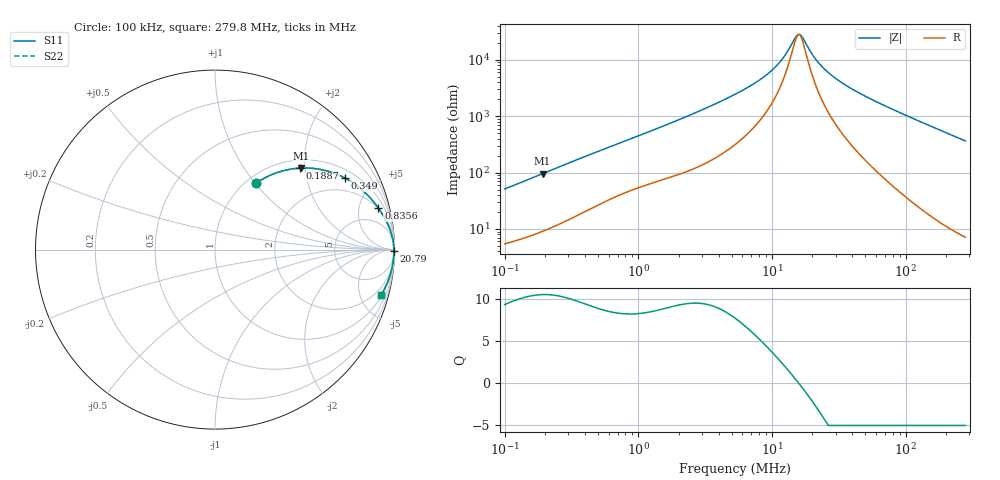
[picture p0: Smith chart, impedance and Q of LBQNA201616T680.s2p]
! LBQNA201616T680  S-PARAMETER MODEL  ( General Type )
! Model Generated by TAIYO YUDEN Corporation (http://www.ty-top.com)
! Version 1.0
! TAIYO YUDEN Control No. 191025NI43SB-FBB
! Copyright(c) 2019 TAIYO YUDEN CO.,LTD. All Rights Reserved.
! Product Description (link to TY-COMPAS)
! https://ds.yuden.co.jp/TYCOMPAS/or/detail?pn=LBQNA201616T680K&u=M
! Products Name : Inductors
! Characteristics :
!  Inductance : 68 uH , SRF(min) : 10 MHz , DC Resistance(max) : 3.9 Ohm
!  Rated Current : Saturation :90 mA , Temp Rise : 110 mA (20 degC)
!  Case Size : 2.0 x 1.6 / 0.079 x 0.063 [mm/inch] , Thickness : 1.6 / 0.063 [mm/inch]
!  (Conditions: Temperature = 25 degC , DC Bias Current/Voltage = 0A / 0V)
! External Node Assignments :
!  1  o---GGG---o  2
! GND o---------o GND
! Frequency Range : 0.1MHz  -  279.750408MHz  [ 402 STEP ]
# MHz S RI R 50
! Freq[MHz].  S11 Real  S11 Imag  S21 Real  S21 Imag  S12 Real  S12 Imag  S22 Real  S22 Imag
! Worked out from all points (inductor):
!   401 points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, 100 kHz to 279.8 MHz, reference 50 ohm
!   read as one part in series: L = 80 uH near 104 kHz
!   highest Q = 10.5 at 192.5 kHz (marker M1), where L = 78.9 uH
!   self-resonance near 15.75 MHz
!   S11 on the Smith chart (normalised r, x): 100 kHz: 1.11, +1.01; 188.7 kHz: 1.18, +1.87; 349 kHz: 1.35, +3.37; 835.6 kHz: 1.92, +7.54; 20.79 MHz: open; 279.8 MHz: 1.14, -7.27
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0.1  0.2294 0.3703  0.7706 -0.3703  0.7706 -0.3703  0.2294 0.3703
0.188687  0.4721 0.4539  0.5279 -0.4539  0.5279 -0.4539  0.4721 0.4539
0.192468  0.4808 0.4544  0.5192 -0.4544  0.5192 -0.4544  0.4808 0.4544
0.349033  0.7221 0.3996  0.2779 -0.3996  0.2779 -0.3996  0.7221 0.3996
0.377863  0.7479 0.385  0.2521 -0.385  0.2521 -0.385  0.7479 0.385
0.835625  0.9108 0.2307  0.0892 -0.2307  0.0892 -0.2307  0.9108 0.2307
1.427803  0.9585 0.1502  0.0415 -0.1502  0.0415 -0.1502  0.9585 0.1502
5.289144  0.9931 0.0402  0.00686 -0.0402  0.00686 -0.0402  0.9931 0.0402
7.710934  0.9951 0.0239  0.00494 -0.0239  0.00494 -0.0239  0.9951 0.0239
10.17991  0.9958 0.0141  0.00415 -0.0141  0.00415 -0.0141  0.9958 0.0141
12.17016  0.9962 0.00827  0.00382 -0.00827  0.00382 -0.00827  0.9962 0.00827
14.84108  0.9964 0.00209  0.00359 -0.00209  0.00359 -0.00209  0.9964 0.00209
15.7513  0.9965 0.00025  0.00354 -0.00025  0.00354 -0.00025  0.9965 0.00025
17.05234  0.9965 -0.0022  0.00349 0.0022  0.00349 0.0022  0.9965 -0.0022
19.9857  0.9965 -0.00718  0.00345 0.00718  0.00345 0.00718  0.9965 -0.00718
20.79473  0.9965 -0.00845  0.00345 0.00845  0.00345 0.00845  0.9965 -0.00845
25.35844  0.9965 -0.015  0.00354 0.015  0.00354 0.015  0.9965 -0.015
32.82031  0.9961 -0.0246  0.00385 0.0246  0.00385 0.0246  0.9961 -0.0246
46.90804  0.9951 -0.0406  0.00488 0.0406  0.00488 0.0406  0.9951 -0.0406
75.51853  0.9917 -0.0703  0.00828 0.0703  0.00828 0.0703  0.9917 -0.0703
148.2617  0.976 -0.1405  0.024 0.1405  0.024 0.1405  0.976 -0.1405
279.7504  0.9254 -0.2531  0.0746 0.2531  0.0746 0.2531  0.9254 -0.2531
